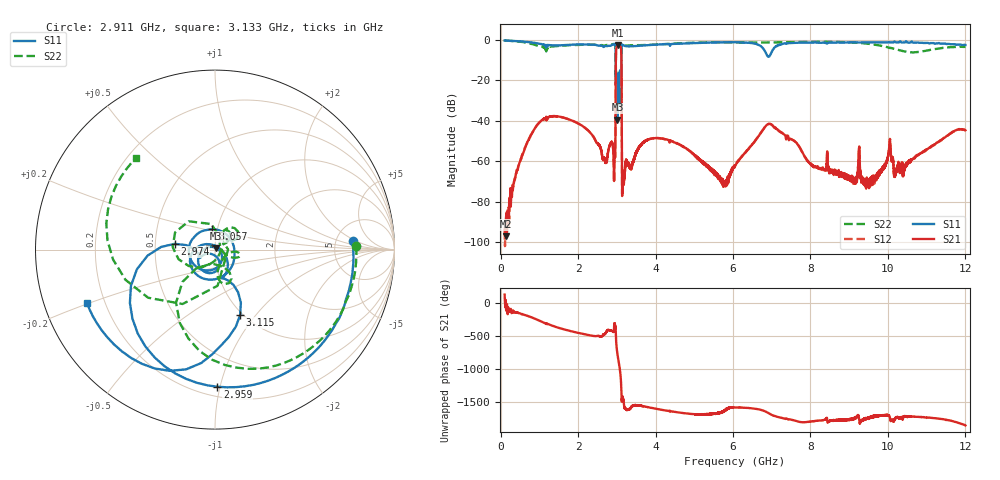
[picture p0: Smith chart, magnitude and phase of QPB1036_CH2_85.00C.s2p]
! TDS: K:\Engsetup\Winsaw\QPB1036_ALL
! Channel 1
! Ports=1 2
! seg 1=100.000000 1100.000000 101
! seg 2=1101.000000 1501.000000 401
! seg 3=1502.000000 2502.000000 101
! seg 4=2503.000000 3803.000000 1301
! seg 5=3804.000000 5004.000000 121
! seg 6=5005.000000 6005.000000 1001
! seg 7=6006.000000 8406.000000 241
! seg 8=8407.000000 10607.000000 2201
! seg 9=10608.000000 12008.000000 141
! Points=5609
! FailCode=0
! Topology=ALL_SE(12)
!VNA Cal loaded =QPB1036_ALL_85C
!PS1(V)= 5.000
!PS(mA)= 0.500
!PS2(V)= 0.630
!PS(mA)= -0.100
!PS3(V)= 1.170
!PS(mA)= 0.100
!PS4(V)= 0.630
!PS(mA)= -0.100
!Temp (C)= 85.00
# MHz S DB R 50
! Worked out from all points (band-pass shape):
!   5609 points, 100 MHz to 12.01 GHz, reference 50 ohm
!   highest |S21| = -2.59 dB at 3.031 GHz (marker M1); lowest = -97.2 dB at 130 MHz (marker M2)
!   |S21| within 3 dB of the highest: 2.982 GHz to 3.113 GHz (131.6 MHz wide, 4.32 % of centre)
!   lowest |S11| = -39.5 dB at 3.015 GHz (marker M3), VSWR 1.02, Z = 50.5 + j0.928 ohm
!   |S11| at or under -10 dB: 2.973 GHz to 3.114 GHz (141 MHz wide, 4.63 % of centre)
!   |S22| runs from -29.6 to -0.3 dB; largest |S21 - S12| = 0.0081
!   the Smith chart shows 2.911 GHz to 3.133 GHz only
!   S11 on the Smith chart (normalised r, x): 2.911 GHz: 7.21, +1.70; 2.959 GHz: 0.27, -0.98; 2.974 GHz: 0.63, +0.04; 3.057 GHz: 0.95, +0.22; 3.115 GHz: 0.97, -0.83; 3.133 GHz: 0.13, -0.20
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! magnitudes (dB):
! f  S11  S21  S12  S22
! 100 MHz  -0.3  -94.0  -94.6  -0.3
! 130 MHz  -0.3  -97.2  -89.3  -0.3
! 1.122 GHz  -2.4  -39.1  -39.0  -3.6
! 2.092 GHz  -2.3  -42.4  -42.4  -2.5
! 2.911 GHz  -2.3  -55.9  -55.9  -2.1
! 2.959 GHz  -2.3  -56.2  -56.0  -3.0
! 2.974 GHz  -12.9  -11.5  -11.5  -13.9
! 3.015 GHz  -39.5  -2.8  -2.8  -19.6
! 3.031 GHz  -18.3  -2.6  -2.6  -27.6
! 3.057 GHz  -18.8  -2.9  -2.9  -15.8
! 3.094 GHz  -22.4  -3.4  -3.4  -18.6
! 3.115 GHz  -8.2  -6.7  -6.7  -12.5
! 3.133 GHz  -2.2  -70.1  -68.8  -3.4
! 3.16 GHz  -2.6  -66.0  -66.6  -3.1
! 4.074 GHz  -2.3  -48.7  -48.6  -2.3
! 6.056 GHz  -1.2  -62.5  -61.9  -1.3
! 6.996 GHz  -6.2  -41.9  -41.9  -1.3
! 8.046 GHz  -1.3  -61.7  -61.9  -1.0
! 9.497 GHz  -1.3  -71.6  -71.0  -1.9
! 10.02 GHz  -1.1  -56.0  -56.0  -3.8
! 10.19 GHz  -1.0  -66.1  -66.6  -4.5
! 12.01 GHz  -2.5  -44.7  -44.8  -3.5
